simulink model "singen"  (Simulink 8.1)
settings: Solver=ode5  StartTime=0.0  StopTime=t_sim  FixedStep=0.001  RelTol=1e-3
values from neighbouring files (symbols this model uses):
  a_exsys = 0.3970    (= 0.397)    [sinsyn.m]
  b_exsys = 0.0900    (= 0.09)    [sinsyn.m]
  d = machine(9,1)    [sinsyn.m]
  deltao = angle(eq1)    [sinsyn.m]
  eb = input('infinite bus voltage''\n')    [sinsyn.m]
  edo1 = -(xq-xq1)*iqo    [sinsyn.m]
  efdmax = 1    [sinsyn.m]
  efdmin = -1    [sinsyn.m]
  efdo = eqo-(xd-xq)*ido    [sinsyn.m]
  eqo1 = efdo+(xd-xd1)*ido    [sinsyn.m]
  exc_choice = 3    [sinsyn.m]
  fhp_st = 0.3    [sinsyn.m]
  fip_st = 0.3    [sinsyn.m]
  flp_st = 0.4    [sinsyn.m]
  gov_choice = 3    [sinsyn.m]
  h = machine(8,1)    [sinsyn.m]
  h1 = input('real part of h parameter''\n')    [sinsyn.m]
  h2 = input('imaginary part of h parameter''\n')    [sinsyn.m]
  k_ht = 20    [sinsyn.m]
  k_st = 20    [sinsyn.m]
  ka1 = 400.0    (= 400)    [sinsyn.m]
  ka2 = 400    [sinsyn.m]
  ke_exsys = 1.0    (= 1)    [sinsyn.m]
  kf_exsys = 0.06    [sinsyn.m]
  ks = 0    [sinsyn.m]
  p_down = 0.1    [sinsyn.m]
  p_hydromax = 1.1    [sinsyn.m]
  p_hydromin = 0.1    [sinsyn.m]
  p_steammax = 1.1    [sinsyn.m]
  p_steammin = 0.1    [sinsyn.m]
  p_up = 1.1    [sinsyn.m]
  po = tmo    [sinsyn.m]
  pss_choice = 2    [sinsyn.m]
  ra = machine(1,1)    [sinsyn.m]
  t1 = 1    [sinsyn.m]
  t1_ht = 38.4803    [sinsyn.m]
  t1_st = 0.3    [sinsyn.m]
  t2 = 1    [sinsyn.m]
  t2_ht = 0    [sinsyn.m]
  t2_st = 0    [sinsyn.m]
  t3 = 1    [sinsyn.m]
  t3_ht = 0.5197    [sinsyn.m]
  t3_st = 0.1    [sinsyn.m]
  t4 = 1    [sinsyn.m]
  ta1 = 0.0200    (= 0.02)    [sinsyn.m]
  ta2 = 0.025    [sinsyn.m]
  tb_exsys = 10    [sinsyn.m]
  tc_exsys = 1.0000    (= 1)    [sinsyn.m]
  tch_st = 0.3    [sinsyn.m]
  tco_st = 0.4    [sinsyn.m]
  tdo1 = machine(6,1)    [sinsyn.m]
  te_exsys = 1.0000    (= 1)    [sinsyn.m]
  tf_exsys = 1.0000    (= 1)    [sinsyn.m]
  tmo = eqo1*iqo+edo1*ido+(xd1-xq1)*ido*iqo    [sinsyn.m]
  tqo1 = machine(7,1)    [sinsyn.m]
  tr_exsys = 0.0100    (= 0.01)    [sinsyn.m]
  trh_st = 8    [sinsyn.m]
  tw = 0    [sinsyn.m]
  tw_ht = 1    [sinsyn.m]
  vg = abs(vgc)    [sinsyn.m]
  vrefo = 0    [sinsyn.m]
  vrmax = 1    [sinsyn.m]
  vrmin = -1    [sinsyn.m]
  vs = 0    [sinsyn.m]
  vsmax = 1    [sinsyn.m]
  vsmin = -1    [sinsyn.m]
  wb = 2*pi*f    [sinsyn.m]
  wref = 2*pi*f    [sinsyn.m]
  xd = machine(3,1)    [sinsyn.m]
  xd1 = machine(5,1)    [sinsyn.m]
  xq = machine(2,1)    [sinsyn.m]
  xq1 = machine(4,1)    [sinsyn.m]
  zi = input('imaginary part of z parameter''\n')    [sinsyn.m]
  zr = input('real part of z parameter''\n')    [sinsyn.m]
undefined symbols (not defined in the file or in its folder): A, alpha, delb_distrb_time, eb_distrb_time, eb_final, eb_initial, h1af, h1f, h2af, h2f, omega, phi, tf1, tf2, tm_distrb_time, tm_final, tm_initial, vref_distrb_time, vref_final, vref_initial, wref_distrb_time, wref_final, wref_initial, ziaf, zif, zraf, zrf
libraries: simulink_extras x13

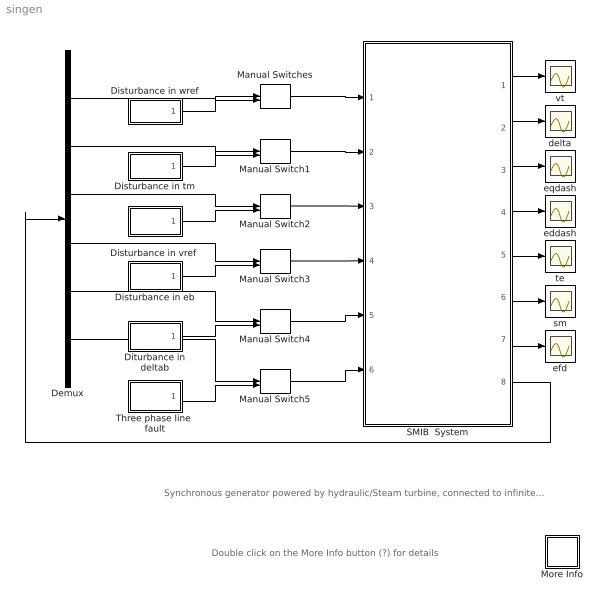
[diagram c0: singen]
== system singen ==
  note: Synchronous generator powered by hydraulic/Steam turbine, connected to infinite bus with excitation , governor systems and PSS.
  note: Double click on the More Info button (?) for details
  Demux : Demux  Outputs=6
  Disturbance in eb : Subsystem
  Disturbance in tm : Subsystem
  "Disturbance in vref " : Subsystem
  Disturbance in wref : Subsystem
  Diturbance in deltab : Subsystem
  Manual Switch{1,3..5} (4 alike) : ManualSwitch
  Manual Switch2 : ManualSwitch  CurrentSetting=0
  Manual Switches : ManualSwitch
  More Info : Subsystem
  SMIB  System : Subsystem
  Three phase line  fault : Subsystem
  delta : Scope
  eddash : Scope
  efd : Scope
  eqdash : Scope
  sm : Scope
  te : Scope
  vt : Scope
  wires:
  SMIB  System/1(vt) -> vt/1
  SMIB  System/3(eqdash) -> eqdash/1
  SMIB  System/4(eddash) -> eddash/1
  SMIB  System/5(te) -> te/1
  SMIB  System/6(sm) -> sm/1
  SMIB  System/7(efd) -> efd/1
  SMIB  System/2(delta) -> delta/1
  Manual Switches/1 -> SMIB  System/1(wref)
  Manual Switch1/1 -> SMIB  System/2(tm)
  Manual Switch2/1 -> SMIB  System/3(vref)
  Manual Switch3/1 -> SMIB  System/4(eb_magnitude)
  Manual Switch4/1 -> SMIB  System/5(eb_angle)
  Manual Switch5/1 -> SMIB  System/6(zh_param)
  SMIB  System/8(ini. cond) -> Demux/1
  Three phase line  fault/1(zh) -> Manual Switch5/2
  Demux/1 -> Manual Switches/1
  Demux/2 -> Manual Switch1/1
  Demux/3 -> Manual Switch2/1
  Demux/4 -> Manual Switch3/1
  Demux/5 -> Manual Switch4/1
  Demux/6 -> Manual Switch5/1
  Disturbance in wref/1(wref) -> Manual Switches/2
  Disturbance in tm/1(tm) -> Manual Switch1/2
  "Disturbance in vref "/1(vref) -> Manual Switch2/2
  Disturbance in eb/1(eb) -> Manual Switch3/2
  Diturbance in deltab/1(deltab) -> Manual Switch4/2

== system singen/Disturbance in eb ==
  eb_in : Step  Time=eb_distrb_time  Before=eb_initial  After=eb_final  SampleTime=0
  eb : Outport
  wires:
  eb_in/1 -> eb/1

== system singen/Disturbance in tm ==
  tm_in : Step  Time=tm_distrb_time  Before=tm_initial  After=tm_final  SampleTime=0
  tm : Outport
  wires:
  tm_in/1 -> tm/1

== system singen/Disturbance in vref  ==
  vref_in : Step  Time=vref_distrb_time  Before=vref_initial  After=vref_final  SampleTime=0
  vref : Outport
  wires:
  vref_in/1 -> vref/1

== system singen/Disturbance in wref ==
  wref_in : Step  Time=wref_distrb_time  Before=wref_initial  After=wref_final  SampleTime=0
  wref : Outport
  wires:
  wref_in/1 -> wref/1

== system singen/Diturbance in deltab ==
  Clock8 : Clock
  Constant25 : Constant  Value=0
  Switch8 : Switch  Threshold=delb_distrb_time
  infbus_angle : Subsystem
  deltab : Outport
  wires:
  infbus_angle/1(del_infb) -> Switch8/1
  Clock8/1 -> Switch8/2
  Switch8/1 -> deltab/1
  Constant25/1 -> Switch8/3

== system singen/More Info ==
  note: Synchronous generator powered by hydraulic/Steam turbine, connected to infinite bus with excitation , governor systems and PSS.
  note: 1. Run the file " sinsyn.m " by typing sinsyn at the command window. Enter the data prompted from the key board.
  note: 2. Start the Simulation.
  note: 6. double click any scope to see the variations of the respective quantitiy
  note: Simulation without disturbance :
  note: In this case all the manual switches are set to its upper input terminal.
  note: Simulation with disturbance :
  note: 3. Double click any scope to see the variations of the respective quantitiy. Since there is no disturbance , all the quantities remain constant with time.
  note: 4. To create a particular disturbance the manual switches are to be set to its lower input terminal. Then double click the appropriate disturbance icon to feed the disturbance data.
  note: (After double clicking appropriate disturbance icon ,use help buton for details regarding disturbance)
  note: 5. Start the Simulation.

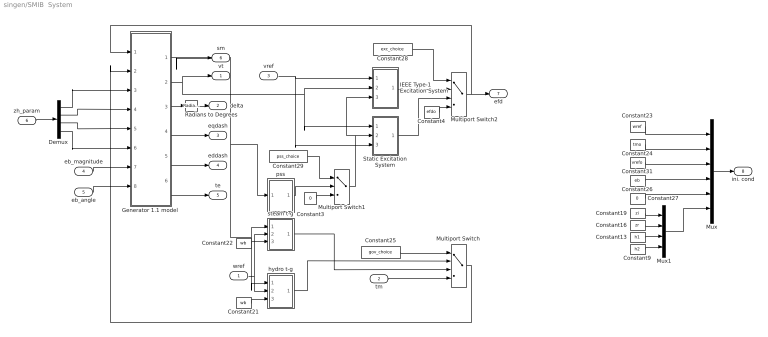
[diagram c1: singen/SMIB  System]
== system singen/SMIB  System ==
  wref : Inport
  tm : Inport  Port=2
  vref : Inport  Port=3
  eb_magnitude : Inport  Port=4
  eb_angle : Inport  Port=5
  zh_param : Inport  Port=6
  Constant13 : Constant  Value=h1
  Constant16 : Constant  Value=zr
  Constant19 : Constant  Value=zi
  Constant21 : Constant  Value=wb
  Constant22 : Constant  Value=wb
  Constant23 : Constant  Value=wref
  Constant24 : Constant  Value=tmo
  Constant25 : Constant  Value=gov_choice
  Constant26 : Constant  Value=eb
  Constant27 : Constant  Value=0
  Constant28 : Constant  Value=exc_choice
  Constant29 : Constant  Value=pss_choice
  Constant3 : Constant  Value=0
  Constant31 : Constant  Value=vrefo
  Constant4 : Constant  Value=efdo
  Constant9 : Constant  Value=h2
  Demux : Demux
  "Generator 1.1 model " : Subsystem
  IEEE Type-1 Excitation System : Subsystem
  Multiport Switch : MultiPortSwitch
  Multiport Switch1 : MultiPortSwitch  Inputs=2
  Multiport Switch2 : MultiPortSwitch
  Mux : Mux  Inputs=6
  Mux1 : Mux
  Radians to Degrees : simulink_extras/Transformations/Radians to Degrees
  Static Excitation System : Subsystem
  hydro t-g : Subsystem
  pss : Subsystem
  steam t-g : Subsystem
  vt : Outport
  delta : Outport  Port=2
  eqdash : Outport  Port=3
  eddash : Outport  Port=4
  te : Outport  Port=5
  sm : Outport  Port=6
  efd : Outport  Port=7
  ini. cond : Outport  Port=8
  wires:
  "Generator 1.1 model "/1(sm) -> pss/1(sm), steam t-g/1(sm), hydro t-g/1(sm), sm/1
  eb_magnitude/1 -> "Generator 1.1 model "/7(eb)
  "Generator 1.1 model "/3(delta) -> Radians to Degrees/1
  "Generator 1.1 model "/2(vt) -> vt/1, IEEE Type-1 Excitation System/2(vt), Static Excitation System/1(vt)
  vref/1 -> IEEE Type-1 Excitation System/1(vrefo), Static Excitation System/3(vrefo)
  eb_angle/1 -> "Generator 1.1 model "/8(ang_infb)
  zh_param/1 -> Demux/1
  Demux/1 -> "Generator 1.1 model "/3(zi)
  Demux/2 -> "Generator 1.1 model "/4(zr)
  Demux/3 -> "Generator 1.1 model "/5(h1)
  Demux/4 -> "Generator 1.1 model "/6(h2)
  "Generator 1.1 model "/4(eq1) -> eqdash/1
  "Generator 1.1 model "/5(ed1) -> eddash/1
  "Generator 1.1 model "/6(te) -> te/1
  IEEE Type-1 Excitation System/1(efd) -> Multiport Switch2/2
  Static Excitation System/1(efd) -> Multiport Switch2/3
  Constant4/1 -> Multiport Switch2/4
  Multiport Switch1/1 -> IEEE Type-1 Excitation System/3(vs), Static Excitation System/2(vs)
  Multiport Switch2/1 -> "Generator 1.1 model "/1(efd), efd/1
  Constant21/1 -> hydro t-g/3(wb)
  Constant22/1 -> steam t-g/3(wb)
  wref/1 -> hydro t-g/2(wref), steam t-g/2(wref)
  Multiport Switch/1 -> "Generator 1.1 model "/2(tm)
  tm/1 -> Multiport Switch/4
  Constant3/1 -> Multiport Switch1/3
  pss/1(vs) -> Multiport Switch1/2
  Radians to Degrees/1 -> delta/1
  Constant9/1 -> Mux1/4
  Constant19/1 -> Mux1/1
  Constant16/1 -> Mux1/2
  Constant13/1 -> Mux1/3
  Constant23/1 -> Mux/1
  Constant24/1 -> Mux/2
  Constant26/1 -> Mux/4
  Constant27/1 -> Mux/5
  Mux1/1 -> Mux/6
  Mux/1 -> ini. cond/1
  Constant28/1 -> Multiport Switch2/1
  Constant31/1 -> Mux/3
  Constant25/1 -> Multiport Switch/1
  Constant29/1 -> Multiport Switch1/1
  hydro t-g/1(pm) -> Multiport Switch/2
  steam t-g/1(pm) -> Multiport Switch/3

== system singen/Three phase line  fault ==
  Subsystem1 : Subsystem
  zh : Outport
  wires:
  Subsystem1/1(zh) -> zh/1

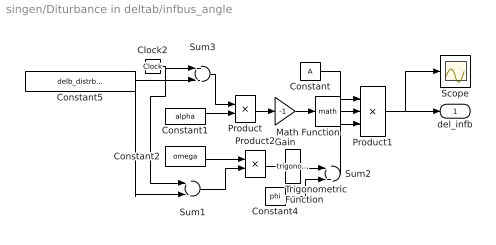
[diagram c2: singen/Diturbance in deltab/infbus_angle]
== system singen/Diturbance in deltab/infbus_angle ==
  Clock2 : Clock
  Constant : Constant  Value=A
  Constant1 : Constant  Value=alpha
  Constant2 : Constant  Value=omega
  Constant4 : Constant  Value=phi
  Constant5 : Constant  Value=delb_distrb_time
  Gain : Gain  Gain=-1
  Math Function : Math
  Product : Product
  Product1 : Product  Inputs=3
  Product2 : Product
  Scope : Scope
  Sum1 : Sum  Inputs=+-
  Sum2 : Sum
  Sum3 : Sum  Inputs=+-
  Trigonometric Function : Trigonometry
  del_infb : Outport
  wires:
  Constant1/1 -> Product/2
  Product/1 -> Gain/1
  Gain/1 -> Math Function/1
  Constant/1 -> Product1/1
  Math Function/1 -> Product1/2
  Sum1/1 -> Product2/2
  Product2/1 -> Trigonometric Function/1
  Trigonometric Function/1 -> Sum2/1
  Constant4/1 -> Sum2/2
  Sum2/1 -> Product1/3
  Sum3/1 -> Product/1
  Constant5/1 -> Sum3/2, Sum1/2
  Clock2/1 -> Sum3/1, Sum1/1
  Constant2/1 -> Product2/1
  Product1/1 -> del_infb/1, Scope/1

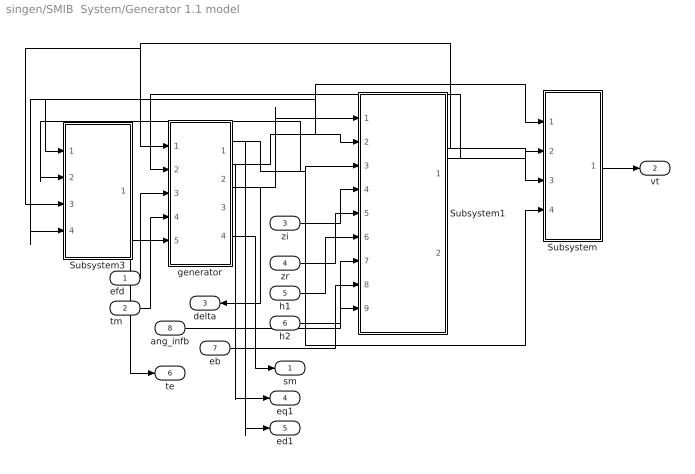
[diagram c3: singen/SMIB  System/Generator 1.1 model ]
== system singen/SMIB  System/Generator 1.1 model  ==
  efd : Inport
  tm : Inport  Port=2
  zi : Inport  Port=3
  zr : Inport  Port=4
  h1 : Inport  Port=5
  h2 : Inport  Port=6
  eb : Inport  Port=7
  ang_infb : Inport  Port=8
  Subsystem : Subsystem
  Subsystem1 : Subsystem
  Subsystem3 : Subsystem
  generator : Subsystem
  sm : Outport
  vt : Outport  Port=2
  delta : Outport  Port=3
  eq1 : Outport  Port=4
  ed1 : Outport  Port=5
  te : Outport  Port=6
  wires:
  ang_infb/1 -> Subsystem1/9(ang_infb)
  efd/1 -> generator/3(efd)
  eb/1 -> Subsystem1/8(eb)
  Subsystem1/1(id) -> Subsystem/2(id), generator/2(id), Subsystem3/1(id)
  generator/4(sm) -> sm/1
  zi/1 -> Subsystem1/4(zi)
  zr/1 -> Subsystem1/5(zr)
  h1/1 -> Subsystem1/6(h1)
  h2/1 -> Subsystem1/7(h2)
  generator/3(delta) -> Subsystem1/1(delta), delta/1
  tm/1 -> generator/4(pm)
  generator/2(eq1) -> Subsystem1/2(eq1), Subsystem/1(eq1), Subsystem3/4(eq1), eq1/1
  generator/1(ed1) -> Subsystem1/3(ed1), Subsystem/4(ed1), Subsystem3/2(ed1), ed1/1
  Subsystem1/2(iq) -> Subsystem/3(iq), generator/1(iq), Subsystem3/3(iq)
  Subsystem3/1(te) -> generator/5(Te), te/1
  Subsystem/1(vt) -> vt/1

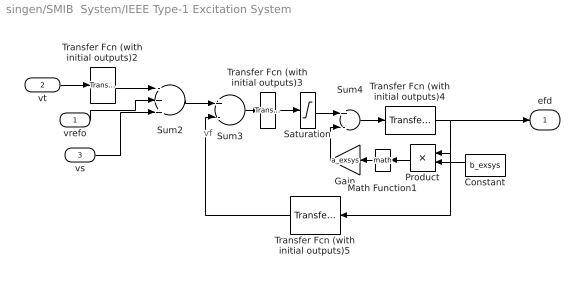
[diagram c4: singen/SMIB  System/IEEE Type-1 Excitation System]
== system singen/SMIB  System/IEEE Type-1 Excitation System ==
  note: vf
  vrefo : Inport
  vt : Inport  Port=2
  vs : Inport  Port=3
  Constant : Constant  Value=b_exsys
  Gain : Gain  Gain=a_exsys
  Math Function1 : Math
  Product : Product
  Saturation : Saturate  UpperLimit=vrmax  LowerLimit=vrmin
  Sum2 : Sum  Inputs=-++
  Sum3 : Sum  Inputs=+-
  Sum4 : Sum  Inputs=+-
  Transfer Fcn (with initial outputs)2 : simulink_extras/Additional Linear/Transfer Fcn (with initial outputs)  N=[1]  D="[tr_exsys  1]"  Y0=vg  U0=vg
  Transfer Fcn (with initial outputs)3 : simulink_extras/Additional Linear/Transfer Fcn (with initial outputs)  N=[ka1]  D="[ta1  1]"  Y0=ka1*((vrefo-vg+vs))  U0=(vrefo-vg+vs)
  Transfer Fcn (with initial outputs)4 : simulink_extras/Additional Linear/Transfer Fcn (with initial outputs)  N=[1]  D="[te_exsys  ke_exsys]"  Y0=(ka1*((vrefo-vg+vs))-a_exsys*exp(b_exsys*efdo))*1/ke_exsys  U0=ka1*((vrefo-vg+vs))-a_exsys*exp(b_exsys*efdo)
  Transfer Fcn (with initial outputs)5 : simulink_extras/Additional Linear/Transfer Fcn (with initial outputs)  N=[kf_exsys,0]  D=[tf_exsys,1]  Y0=0  U0=efdo
  efd : Outport
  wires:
  Constant/1 -> Product/2
  Product/1 -> Math Function1/1
  Math Function1/1 -> Gain/1
  Saturation/1 -> Sum4/1
  Transfer Fcn (with initial outputs)3/1 -> Saturation/1
  Sum2/1 -> Sum3/1
  Transfer Fcn (with initial outputs)5/1 -> Sum3/2
  Gain/1 -> Sum4/2
  Sum3/1 -> Transfer Fcn (with initial outputs)3/1
  Sum4/1 -> Transfer Fcn (with initial outputs)4/1
  vs/1 -> Sum2/3
  vrefo/1 -> Sum2/2
  vt/1 -> Transfer Fcn (with initial outputs)2/1
  Transfer Fcn (with initial outputs)4/1 -> Product/1, Transfer Fcn (with initial outputs)5/1, efd/1
  Transfer Fcn (with initial outputs)2/1 -> Sum2/1

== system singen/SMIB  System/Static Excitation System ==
  vt : Inport
  vs : Inport  Port=2
  vrefo : Inport  Port=3
  Saturation : Saturate  UpperLimit=efdmax  LowerLimit=efdmin
  Sum1 : Sum  Inputs=-++
  Transfer Fcn (with initial outputs) : simulink_extras/Additional Linear/Transfer Fcn (with initial outputs)  N=[ka2]  D=[ta2,1]  Y0=ka2*(vrefo-vg+vs)  U0=(vrefo-vg+vs)
  Transfer Fcn (with initial outputs)1 : simulink_extras/Additional Linear/Transfer Fcn (with initial outputs)  N=[tc_exsys,1]  D=[tb_exsys,1]  Y0=(vrefo-vg+vs)  U0=(vrefo-vg+vs)
  efd : Outport
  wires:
  Transfer Fcn (with initial outputs)/1 -> Saturation/1
  Sum1/1 -> Transfer Fcn (with initial outputs)1/1
  Transfer Fcn (with initial outputs)1/1 -> Transfer Fcn (with initial outputs)/1
  vt/1 -> Sum1/1
  vs/1 -> Sum1/2
  vrefo/1 -> Sum1/3
  Saturation/1 -> efd/1

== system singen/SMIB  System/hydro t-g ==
  sm : Inport
  wref : Inport  Port=2
  wb : Inport  Port=3
  del_omega1 : Subsystem
  hydro governor : Subsystem
  hydro turbine : Subsystem
  pm : Outport
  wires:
  wb/1 -> del_omega1/3(wb)
  sm/1 -> del_omega1/1(sm)
  del_omega1/1(del -omega) -> hydro governor/1(del_omega)
  hydro turbine/1(pm) -> pm/1
  hydro governor/1(pgv) -> hydro turbine/1(pgv)
  wref/1 -> del_omega1/2(wref)

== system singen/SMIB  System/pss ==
  sm : Inport
  Display : Display
  Saturation : Saturate  UpperLimit=vsmax  LowerLimit=vsmin
  Transfer Fcn : TransferFcn  Numerator=[tw,0]  Denominator=[tw,1]
  Transfer Fcn1 : TransferFcn  Numerator=[ks*t1*t3,ks*(t1+t3),ks]  Denominator=[t4*t2,(t2+t4),1]
  vs : Outport
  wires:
  Saturation/1 -> Display/1, vs/1
  Transfer Fcn1/1 -> Saturation/1
  Transfer Fcn/1 -> Transfer Fcn1/1
  sm/1 -> Transfer Fcn/1

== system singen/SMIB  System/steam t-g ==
  sm : Inport
  wref : Inport  Port=2
  wb : Inport  Port=3
  del_omega1 : Subsystem
  governor : Subsystem
  turbine : Subsystem
  pm : Outport
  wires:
  wb/1 -> del_omega1/3(wb)
  wref/1 -> del_omega1/2(wref)
  del_omega1/1(del -omega) -> governor/1(del_omega)
  sm/1 -> del_omega1/1(sm)
  turbine/1(pm) -> pm/1
  governor/1(pgv) -> turbine/1(pgv)

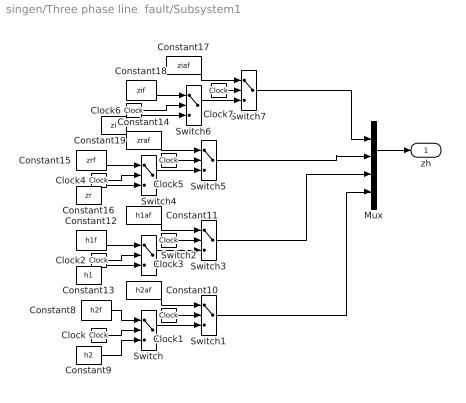
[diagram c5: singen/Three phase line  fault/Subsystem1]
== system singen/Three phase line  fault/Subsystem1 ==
  Clock{,1..7} (8 alike) : Clock
  Constant10 : Constant  Value=h2af
  Constant11 : Constant  Value=h1af
  Constant12 : Constant  Value=h1f
  Constant13 : Constant  Value=h1
  Constant14 : Constant  Value=zraf
  Constant15 : Constant  Value=zrf
  Constant16 : Constant  Value=zr
  Constant17 : Constant  Value=ziaf
  Constant18 : Constant  Value=zif
  Constant19 : Constant  Value=zi
  Constant8 : Constant  Value=h2f
  Constant9 : Constant  Value=h2
  Mux : Mux
  Switch{,2,4,6} (4 alike) : Switch  Threshold=tf1
  Switch{1,3,5,7} (4 alike) : Switch  Threshold=tf2
  zh : Outport
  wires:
  Mux/1 -> zh/1
  Switch1/1 -> Mux/4
  Switch3/1 -> Mux/3
  Switch5/1 -> Mux/2
  Switch7/1 -> Mux/1
  Constant19/1 -> Switch6/3
  Constant17/1 -> Switch7/1
  Clock7/1 -> Switch7/2
  Switch6/1 -> Switch7/3
  Constant18/1 -> Switch6/1
  Clock6/1 -> Switch6/2
  Constant16/1 -> Switch4/3
  Constant14/1 -> Switch5/1
  Clock5/1 -> Switch5/2
  Switch4/1 -> Switch5/3
  Constant15/1 -> Switch4/1
  Clock4/1 -> Switch4/2
  Constant13/1 -> Switch2/3
  Constant11/1 -> Switch3/1
  Clock3/1 -> Switch3/2
  Switch2/1 -> Switch3/3
  Constant12/1 -> Switch2/1
  Clock2/1 -> Switch2/2
  Constant10/1 -> Switch1/1
  Clock1/1 -> Switch1/2
  Switch/1 -> Switch1/3
  Constant9/1 -> Switch/3
  Constant8/1 -> Switch/1
  Clock/1 -> Switch/2

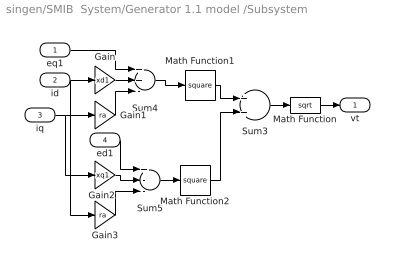
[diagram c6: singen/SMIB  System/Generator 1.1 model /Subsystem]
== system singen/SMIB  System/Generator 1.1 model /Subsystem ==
  eq1 : Inport
  id : Inport  Port=2
  iq : Inport  Port=3
  ed1 : Inport  Port=4
  Gain : Gain  Gain=xd1
  Gain1 : Gain  Gain=ra
  Gain2 : Gain  Gain=xq1
  Gain3 : Gain  Gain=ra
  Math Function : Math  Operator=sqrt
  Math Function1 : Math  Operator=square
  Math Function2 : Math  Operator=square
  Sum3 : Sum
  Sum4 : Sum  Inputs=++-
  Sum5 : Sum  Inputs=+--
  vt : Outport
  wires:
  Sum5/1 -> Math Function2/1
  Sum4/1 -> Math Function1/1
  Sum3/1 -> Math Function/1
  Math Function/1 -> vt/1
  eq1/1 -> Sum4/1
  Gain/1 -> Sum4/2
  Gain1/1 -> Sum4/3
  Math Function1/1 -> Sum3/1
  Math Function2/1 -> Sum3/2
  ed1/1 -> Sum5/1
  Gain2/1 -> Sum5/2
  Gain3/1 -> Sum5/3
  iq/1 -> Gain1/1, Gain2/1
  id/1 -> Gain/1, Gain3/1

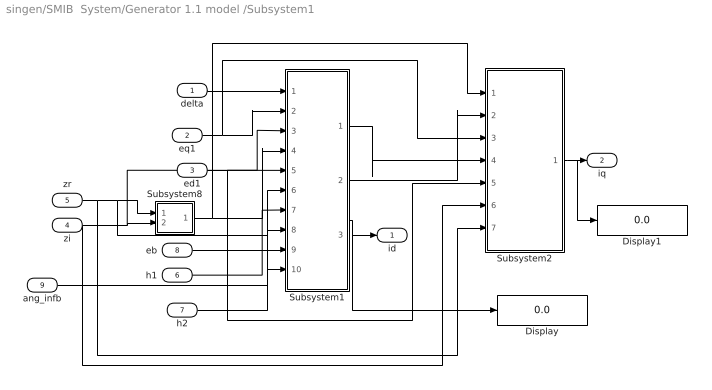
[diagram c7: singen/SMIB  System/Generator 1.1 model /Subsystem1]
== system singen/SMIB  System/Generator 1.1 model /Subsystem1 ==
  delta : Inport
  eq1 : Inport  Port=2
  ed1 : Inport  Port=3
  zi : Inport  Port=4
  zr : Inport  Port=5
  h1 : Inport  Port=6
  h2 : Inport  Port=7
  eb : Inport  Port=8
  ang_infb : Inport  Port=9
  Display : Display
  Display1 : Display
  Subsystem1 : Subsystem
  Subsystem2 : Subsystem
  Subsystem8 : Subsystem
  id : Outport
  iq : Outport  Port=2
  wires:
  ang_infb/1 -> Subsystem1/10(ang_infb)
  eb/1 -> Subsystem1/9(eb)
  delta/1 -> Subsystem1/1(delta)
  Subsystem1/2(f1) -> Subsystem2/2(f1)
  Subsystem1/1(f2) -> Subsystem2/4(f2)
  eq1/1 -> Subsystem1/2(eq1), Subsystem2/3(eq1)
  ed1/1 -> Subsystem1/3(ed1), Subsystem2/5(ed1)
  h1/1 -> Subsystem1/7(h1)
  h2/1 -> Subsystem1/8(h2)
  zr/1 -> Subsystem8/1(zr), Subsystem1/6(zr), Subsystem2/7(zr)
  zi/1 -> Subsystem8/2(zi), Subsystem1/5(zi), Subsystem2/6(zi)
  Subsystem8/1(det) -> Subsystem1/4(det), Subsystem2/1(det)
  Subsystem1/3(id) -> id/1, Display/1
  Subsystem2/1(iq) -> iq/1, Display1/1

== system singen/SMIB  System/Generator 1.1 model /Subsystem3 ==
  note: id
  note: iq
  id : Inport
  ed1 : Inport  Port=2
  iq : Inport  Port=3
  eq1 : Inport  Port=4
  Display : Display
  Gain : Gain  Gain=xd1-xq1
  Product : Product
  Product1 : Product
  Product2 : Product
  Sum : Sum  Inputs=+++
  te : Outport
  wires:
  Sum/1 -> Display/1, te/1
  ed1/1 -> Product/2
  Product/1 -> Sum/1
  Product1/1 -> Sum/2
  id/1 -> Product/1, Product2/1
  Product2/1 -> Gain/1
  Gain/1 -> Sum/3
  eq1/1 -> Product1/2
  iq/1 -> Product1/1, Product2/2

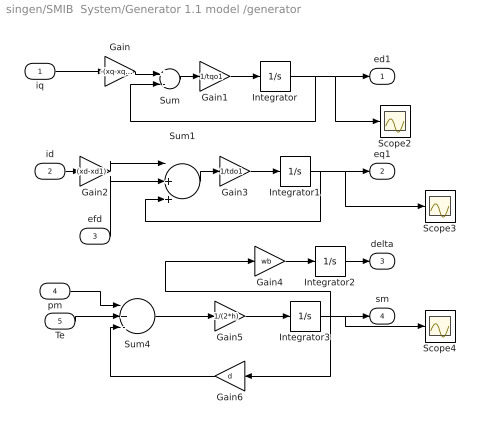
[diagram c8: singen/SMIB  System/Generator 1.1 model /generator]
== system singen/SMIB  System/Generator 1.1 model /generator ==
  iq : Inport
  id : Inport  Port=2
  efd : Inport  Port=3
  pm : Inport  Port=4
  Te : Inport  Port=5
  Gain : Gain  Gain=-(xq-xq1)
  Gain1 : Gain  Gain=1/tqo1
  Gain2 : Gain  Gain=(xd-xd1)
  Gain3 : Gain  Gain=1/tdo1
  Gain4 : Gain  Gain=wb
  Gain5 : Gain  Gain=1/(2*h)
  Gain6 : Gain  Gain=d
  Integrator : Integrator  InitialCondition=edo1
  Integrator1 : Integrator  InitialCondition=eqo1
  Integrator2 : Integrator  InitialCondition=deltao
  Integrator3 : Integrator
  Scope2 : Scope
  Scope3 : Scope
  Scope4 : Scope
  Sum : Sum  Inputs=+-
  Sum1 : Sum  Inputs=|++-
  Sum4 : Sum  Inputs=|+--
  ed1 : Outport
  eq1 : Outport  Port=2
  delta : Outport  Port=3
  sm : Outport  Port=4
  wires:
  Integrator2/1 -> delta/1
  efd/1 -> Sum1/2
  Integrator/1 -> Sum/2, ed1/1, Scope2/1
  Gain/1 -> Sum/1
  Sum/1 -> Gain1/1
  id/1 -> Gain2/1
  Gain2/1 -> Sum1/1
  Sum1/1 -> Gain3/1
  Gain6/1 -> Sum4/3
  Integrator1/1 -> eq1/1, Scope3/1, Sum1/3
  Integrator3/1 -> Gain4/1, Gain6/1, sm/1, Scope4/1
  pm/1 -> Sum4/1
  Te/1 -> Sum4/2
  Sum4/1 -> Gain5/1
  iq/1 -> Gain/1
  Gain1/1 -> Integrator/1
  Gain3/1 -> Integrator1/1
  Gain4/1 -> Integrator2/1
  Gain5/1 -> Integrator3/1

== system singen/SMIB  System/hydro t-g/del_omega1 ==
  sm : Inport
  wref : Inport  Port=2
  wb : Inport  Port=3
  Constant1 : Constant
  Product1 : Product  Inputs=*/
  Sum : Sum
  Sum1 : Sum  Inputs=-+
  del -omega : Outport
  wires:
  Sum1/1 -> del -omega/1
  Product1/1 -> Sum1/2
  Sum/1 -> Sum1/1
  wb/1 -> Product1/2
  wref/1 -> Product1/1
  sm/1 -> Sum/2
  Constant1/1 -> Sum/1

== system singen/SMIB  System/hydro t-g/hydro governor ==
  del_omega : Inport
  Constant : Constant  Value=po
  Saturation : Saturate  UpperLimit=p_hydromax  LowerLimit=p_hydromin
  Sum : Sum  Inputs=-+
  Transfer Fcn (with initial outputs) : simulink_extras/Additional Linear/Transfer Fcn (with initial outputs)  N=[[k_ht*t2_ht,k_ht]]  D=[t1_ht*t3_ht,(t1_ht+t3_ht),1]  Y0=0  U0=0
  pgv : Outport
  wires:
  Saturation/1 -> pgv/1
  Sum/1 -> Saturation/1
  Constant/1 -> Sum/2
  Transfer Fcn (with initial outputs)/1 -> Sum/1
  del_omega/1 -> Transfer Fcn (with initial outputs)/1

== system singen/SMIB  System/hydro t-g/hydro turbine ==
  pgv : Inport
  Transfer Fcn (with initial outputs)1 : simulink_extras/Additional Linear/Transfer Fcn (with initial outputs)  N=[-tw_ht,1]  D=[.5*tw_ht,1]  Y0=po  U0=po
  pm : Outport
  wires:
  pgv/1 -> Transfer Fcn (with initial outputs)1/1
  Transfer Fcn (with initial outputs)1/1 -> pm/1

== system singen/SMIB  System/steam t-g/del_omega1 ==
  sm : Inport
  wref : Inport  Port=2
  wb : Inport  Port=3
  Constant1 : Constant
  Product1 : Product  Inputs=*/
  Sum : Sum
  Sum1 : Sum  Inputs=-+
  del -omega : Outport
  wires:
  Sum1/1 -> del -omega/1
  Product1/1 -> Sum1/2
  Sum/1 -> Sum1/1
  wb/1 -> Product1/2
  wref/1 -> Product1/1
  sm/1 -> Sum/2
  Constant1/1 -> Sum/1

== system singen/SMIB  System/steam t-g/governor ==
  del_omega : Inport
  Constant : Constant  Value=po
  Gain : Gain  Gain=1/t3_st
  Integrator : Integrator  InitialCondition=po  LimitOutput=on  UpperSaturationLimit=p_steammax  LowerSaturationLimit=p_steammin
  Saturation : Saturate  UpperLimit=p_up  LowerLimit=p_down
  Sum : Sum  Inputs=-+-
  Transfer Fcn (with initial outputs) : simulink_extras/Additional Linear/Transfer Fcn (with initial outputs)  N=[t2_st*k_st,k_st]  D=[t1_st,1]  Y0=0  U0=0
  pgv : Outport
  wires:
  Saturation/1 -> Gain/1
  Sum/1 -> Saturation/1
  Transfer Fcn (with initial outputs)/1 -> Sum/1
  del_omega/1 -> Transfer Fcn (with initial outputs)/1
  Gain/1 -> Integrator/1
  Integrator/1 -> pgv/1, Sum/3
  Constant/1 -> Sum/2

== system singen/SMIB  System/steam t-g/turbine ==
  pgv : Inport
  Gain : Gain  Gain=fhp_st
  Gain1 : Gain  Gain=fip_st
  Gain2 : Gain  Gain=flp_st
  Sum : Sum
  Sum1 : Sum
  Transfer Fcn (with initial outputs) : simulink_extras/Additional Linear/Transfer Fcn (with initial outputs)  N=[1]  D="[tch_st  1]"  Y0=po  U0=po
  Transfer Fcn (with initial outputs)1 : simulink_extras/Additional Linear/Transfer Fcn (with initial outputs)  N=[1]  D="[trh_st  1]"  Y0=po  U0=po
  Transfer Fcn (with initial outputs)2 : simulink_extras/Additional Linear/Transfer Fcn (with initial outputs)  N=[1]  D="[tco_st  1]"  Y0=po  U0=po
  pm : Outport
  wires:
  Gain1/1 -> Sum/1
  Gain/1 -> Sum/2
  Sum/1 -> Sum1/2
  Sum1/1 -> pm/1
  pgv/1 -> Transfer Fcn (with initial outputs)/1
  Gain2/1 -> Sum1/1
  Transfer Fcn (with initial outputs)2/1 -> Gain2/1
  Transfer Fcn (with initial outputs)1/1 -> Gain1/1, Transfer Fcn (with initial outputs)2/1
  Transfer Fcn (with initial outputs)/1 -> Gain/1, Transfer Fcn (with initial outputs)1/1

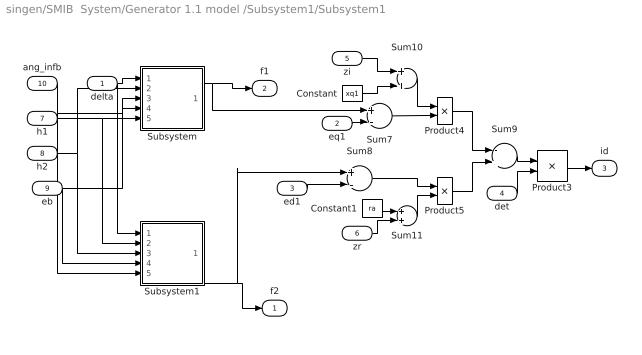
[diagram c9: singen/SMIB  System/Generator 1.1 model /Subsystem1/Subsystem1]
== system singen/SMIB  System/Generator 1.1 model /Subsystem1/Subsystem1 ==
  delta : Inport
  eq1 : Inport  Port=2
  ed1 : Inport  Port=3
  det : Inport  Port=4
  zi : Inport  Port=5
  zr : Inport  Port=6
  h1 : Inport  Port=7
  h2 : Inport  Port=8
  eb : Inport  Port=9
  ang_infb : Inport  Port=10
  Constant : Constant  Value=xq1
  Constant1 : Constant  Value=ra
  Product3 : Product
  Product4 : Product
  Product5 : Product
  Subsystem : Subsystem
  Subsystem1 : Subsystem
  Sum10 : Sum
  Sum11 : Sum
  Sum7 : Sum  Inputs=+-
  Sum8 : Sum  Inputs=+-
  Sum9 : Sum  Inputs=-+
  f2 : Outport
  f1 : Outport  Port=2
  id : Outport  Port=3
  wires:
  ang_infb/1 -> Subsystem1/5(ang_infb), Subsystem/5(ang_infb)
  eb/1 -> Subsystem1/4(eb), Subsystem/4(eb)
  delta/1 -> Subsystem/1(delta), Subsystem1/1(delta)
  Subsystem/1(f1(del)) -> f1/1, Sum7/1
  ed1/1 -> Sum8/2
  Subsystem1/1(f2(del)) -> f2/1, Sum8/1
  Sum9/1 -> Product3/1
  det/1 -> Product3/2
  Product3/1 -> id/1
  eq1/1 -> Sum7/2
  Sum7/1 -> Product4/2
  Product4/1 -> Sum9/1
  Sum10/1 -> Product4/1
  Product5/1 -> Sum9/2
  Sum8/1 -> Product5/1
  Sum11/1 -> Product5/2
  Constant1/1 -> Sum11/1
  Constant/1 -> Sum10/2
  zi/1 -> Sum10/1
  zr/1 -> Sum11/2
  h1/1 -> Subsystem/3(h1), Subsystem1/2(h1)
  h2/1 -> Subsystem1/3(h2), Subsystem/2(h2)

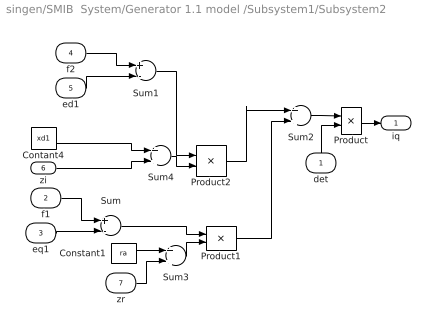
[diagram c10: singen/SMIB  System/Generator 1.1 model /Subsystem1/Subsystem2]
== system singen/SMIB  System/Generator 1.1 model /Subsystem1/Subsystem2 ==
  det : Inport
  f1 : Inport  Port=2
  eq1 : Inport  Port=3
  f2 : Inport  Port=4
  ed1 : Inport  Port=5
  zi : Inport  Port=6
  zr : Inport  Port=7
  Constant1 : Constant  Value=ra
  Contant4 : Constant  Value=xd1
  Product : Product
  Product1 : Product
  Product2 : Product
  Sum : Sum  Inputs=+-
  Sum1 : Sum  Inputs=+-
  Sum2 : Sum
  Sum3 : Sum
  Sum4 : Sum
  iq : Outport
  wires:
  Sum2/1 -> Product/1
  det/1 -> Product/2
  Product/1 -> iq/1
  ed1/1 -> Sum1/2
  f2/1 -> Sum1/1
  Sum1/1 -> Product2/1
  Contant4/1 -> Sum4/1
  Sum4/1 -> Product2/2
  zi/1 -> Sum4/2
  eq1/1 -> Sum/2
  f1/1 -> Sum/1
  Sum/1 -> Product1/1
  Constant1/1 -> Sum3/1
  Sum3/1 -> Product1/2
  zr/1 -> Sum3/2
  Product2/1 -> Sum2/1
  Product1/1 -> Sum2/2

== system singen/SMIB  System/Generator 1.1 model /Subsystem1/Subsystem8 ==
  zr : Inport
  zi : Inport  Port=2
  Constant : Constant  Value=xd1
  Constant2 : Constant  Value=ra
  Constant8 : Constant  Value=xq1
  Fcn : Fcn  Expr=1/u
  Product : Product
  Product2 : Product
  Sum1 : Sum
  Sum2 : Sum
  Sum3 : Sum  Inputs=--
  Sum4 : Sum
  det : Outport
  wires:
  Constant/1 -> Sum1/1
  Sum3/1 -> Fcn/1
  Sum1/1 -> Product2/1
  Constant2/1 -> Sum2/1
  Sum2/1 -> Product/1, Product/2
  Sum4/1 -> Product2/2
  Constant8/1 -> Sum4/1
  Product/1 -> Sum3/2
  Product2/1 -> Sum3/1
  Fcn/1 -> det/1
  zr/1 -> Sum2/2
  zi/1 -> Sum1/2, Sum4/2

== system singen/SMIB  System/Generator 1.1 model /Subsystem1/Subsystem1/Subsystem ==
  delta : Inport
  h2 : Inport  Port=2
  h1 : Inport  Port=3
  eb : Inport  Port=4
  ang_infb : Inport  Port=5
  Product{,1..3} (4 alike) : Product
  Sum : Sum
  Sum1 : Sum  Inputs=+-
  Trigonometric Function1 : Trigonometry  Operator=cos
  Trigonometric Function2 : Trigonometry
  f1(del) : Outport
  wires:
  Trigonometric Function2/1 -> Product1/1
  Trigonometric Function1/1 -> Product/1
  Sum/1 -> f1(del)/1
  Product/1 -> Product2/1
  Product2/1 -> Sum/1
  Product1/1 -> Product3/2
  Product3/1 -> Sum/2
  eb/1 -> Product2/2, Product3/1
  h1/1 -> Product/2
  h2/1 -> Product1/2
  delta/1 -> Sum1/1
  ang_infb/1 -> Sum1/2
  Sum1/1 -> Trigonometric Function1/1, Trigonometric Function2/1

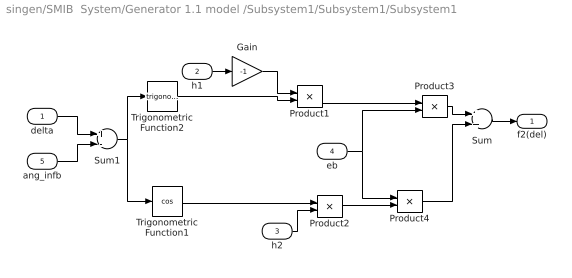
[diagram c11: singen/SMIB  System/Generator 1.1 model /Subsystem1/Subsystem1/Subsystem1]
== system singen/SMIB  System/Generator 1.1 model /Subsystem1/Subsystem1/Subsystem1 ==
  delta : Inport
  h1 : Inport  Port=2
  h2 : Inport  Port=3
  eb : Inport  Port=4
  ang_infb : Inport  Port=5
  Gain : Gain  Gain=-1
  Product{1..4} (4 alike) : Product
  Sum : Sum
  Sum1 : Sum  Inputs=+-
  Trigonometric Function1 : Trigonometry  Operator=cos
  Trigonometric Function2 : Trigonometry
  f2(del) : Outport
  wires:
  Trigonometric Function1/1 -> Product2/1
  Product4/1 -> Sum/2
  Sum/1 -> f2(del)/1
  Product1/1 -> Product3/1
  Product3/1 -> Sum/1
  Product2/1 -> Product4/2
  h2/1 -> Product2/2
  Trigonometric Function2/1 -> Product1/2
  Gain/1 -> Product1/1
  h1/1 -> Gain/1
  eb/1 -> Product4/1, Product3/2
  ang_infb/1 -> Sum1/2
  delta/1 -> Sum1/1
  Sum1/1 -> Trigonometric Function2/1, Trigonometric Function1/1
